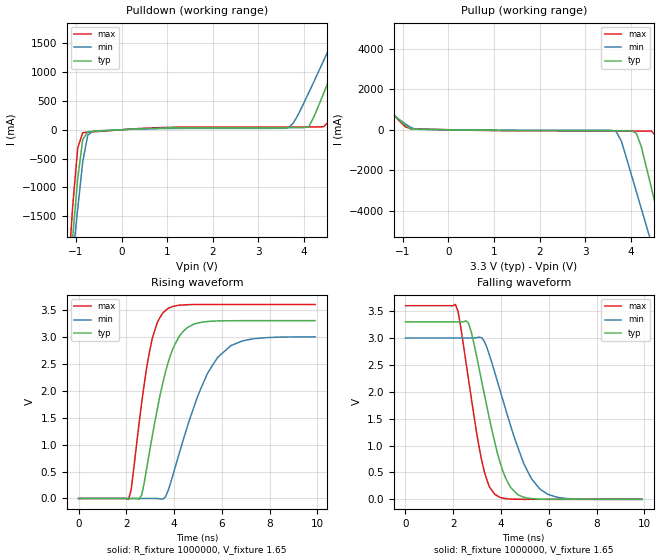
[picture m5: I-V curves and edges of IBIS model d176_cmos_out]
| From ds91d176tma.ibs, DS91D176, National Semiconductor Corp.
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[Model]   d176_cmos_out
Model_type Output
Polarity Non-Inverting
Vref=1.65
Vmeas=1.65
Rref=100000
Cref=15p
C_comp   3.8pF   3.8pF   3.8pF
[Temperature Range]   25   85   -40
[Voltage Range]   3.3   3.0   3.6
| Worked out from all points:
|   slope of the pulldown table from 0 to 0.495 V, typ, clamps not added: 26.1 ohm
|   slope of the pullup table from 0 to 0.495 V, typ, clamps not added: 30.2 ohm
|   rising waveform, R_fixture 1000000, V_fixture 1.65: 20-80 % time 944ps typ, 1.45ns min, 690ps max; typ from 0 V to 3.3 V
|   falling waveform, R_fixture 1000000, V_fixture 1.65: 20-80 % time 994ps typ, 1.32ns min, 770ps max; typ from 3.3 V to 0 V
[Pullup]
|Vtable   (typ)   I(min)   I(max)
-3.58V    5.584A     4.904A     6.677A
-3.36V    5.133A     4.515A     6.127A
-2.92V    4.231A     3.736A     5.028A
-830mV    47.7mA     119mA      49.5mA
3.68V     -43.9mA    -102mA     -62.8mA
4.12V     -179mA     -3.062A    -63.7mA
4.34V     -1.87A     -4.751A    -64.7mA
4.45V     -2.89A     -5.596A    -70.2mA
4.56V     -3.913A    -6.442A    -333mA
4.67V     -4.936A    -7.289A    -1.338A
5V        -8.01A     -9.829A    -5.288A
6.54V     -22.38A    -21.7A     -23.78A
[Pulldown]
|V(pulldown)   I(typ)   I(min)   I(max)
-3.6V     -25.45A    -21.7A     -31.7A
-1.18V    -2.885A    -3.062A    -2.64A
-1.07V    -1.863A    -2.218A    -1.324A
-960mV    -846mA     -1.377A    -316mA
-850mV    -169mA     -556mA     -50.4mA
-740mV    -35.1mA    -96mA      -41.3mA
3.66V     35.1mA     34mA       48mA
4.1V      50.4mA     639mA      48.3mA
4.43V     634mA      1.204A     53.1mA
4.98V     1.734A     2.159A     1.169A
5.31V     2.402A     2.736A     1.981A
7.18V     6.226A     6.035A     6.648A
[Rising Waveform]
R_fixture=1000000
V_fixture=1.65
V_fixture_min=1.5
V_fixture_max=1.8
0s        266pV      738pV      213pV
2.09ns    -71.9nV    38.2nV     -15.7mV
2.2ns     1.32uV     11.2nV     159mV
2.64ns    62.6mV     -12.3nV    1.776V
3.08ns    1.146V     -5.71uV    2.962V
3.74ns    2.51V      135mV      3.526V
4.51ns    3.157V     1.272V     3.595V
5.83ns    3.295V     2.622V     3.6V
6.93ns    3.3V       2.932V     3.6V
9.9ns     3.3V       3V         3.6V
[Falling Waveform]
R_fixture=1000000
V_fixture=1.65
V_fixture_min=1.5
V_fixture_max=1.8
0s        3.3V       3V         3.6V
2.09ns    3.3V       3V         3.622V
2.2ns     3.3V       3V         3.496V
2.64ns    3.276V     3V         2.227V
3.19ns    2.197V     3.006V     725mV
3.74ns    1.061V     2.357V     94.3mV
4.4ns     224mV      1.373V     4.64mV
4.95ns    41mV       669mV      429uV
5.61ns    3.94mV     198mV      1.81uV
9.9ns     -418nV     -6.12uV    203nV
[Ramp]
|   typ   min   max
dV/dt_r   1.98V/0.99ns   1.8V/1.32ns   2.16V/0.69ns
dV/dt_f   1.98V/0.95ns   1.8V/1.31ns   2.16V/0.77ns
R_load=0
|[End   d176_cmos_out
